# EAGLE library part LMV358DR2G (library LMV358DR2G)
Source: Datasheet
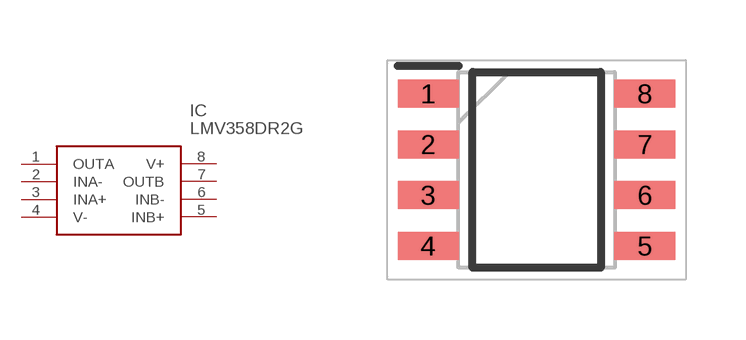
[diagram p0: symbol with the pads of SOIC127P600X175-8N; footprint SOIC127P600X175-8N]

Designator prefix IC

## LMV358DR2G (Height: 1.75mm; Manufacturer_Name: onsemi; Manufacturer_Part_Number: LMV358DR2G; Mouser_Part_Number: 863-LMV358DR2G; Mouser_Price-Stock: https://www.mouser.co.uk/ProductDetail/onsemi/LMV358DR2G?qs=yU2N9dt%252Brfmin4l%252BflhzoQ%3D%3D)  [SOIC127P600X175-8N]
1  OUTA  out
2  INA-  in
3  INA+  in
4  V-
5  INB+  in
6  INB-  in
7  OUTB  out
8  V+

## Footprint SOIC127P600X175-8N (pad centres in mm)
SOIC-8
smd 1.525 x 0.7: 1 -2.712,1.905; 2 -2.712,0.635; 3 -2.712,-0.635; 4 -2.712,-1.905; 5 2.712,-1.905; 6 2.712,-0.635; 7 2.712,0.635; 8 2.712,1.905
